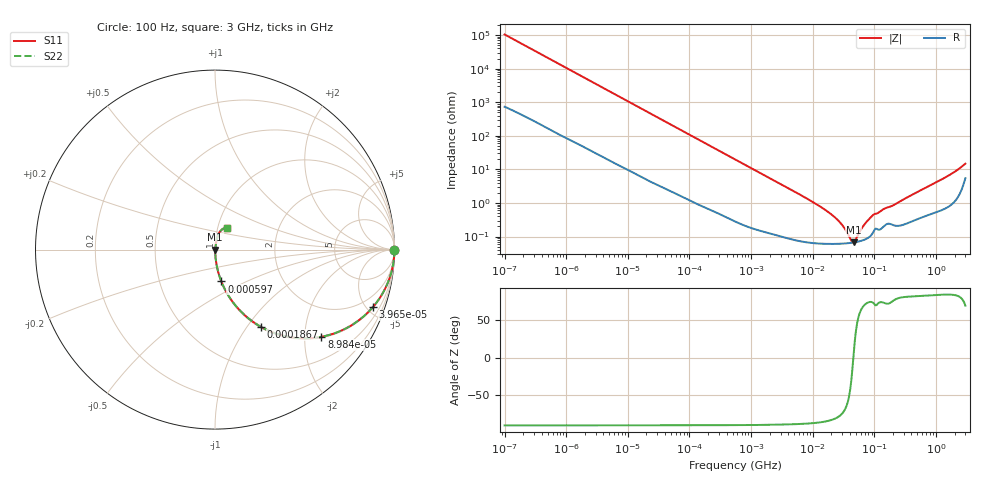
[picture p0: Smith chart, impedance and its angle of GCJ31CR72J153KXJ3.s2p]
!Murata Part Number: GCJ31CR72J153KXJ3
!These Parameters are Measured in Series Mode Connection
!Data Generated on Mar 13, 2026
!  o--ll--o
!Port1  Port2
!  o------o
!Operation Temp=25[degC], DC Bias Voltage=0[V]
!Freq. Start=100[Hz] Stop=3[GHz] 401[Steps]
# Hz S RI R 50
!Freq.(Hz) S11(Real) S11(Imag) S21(Real) S21(Imag) S12(Real) S12(Imag) S22(Real) S22(Imag)
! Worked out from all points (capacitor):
!   401 points, 100 Hz to 3 GHz, reference 50 ohm
!   read as one part in series: C = 15.2 nF near 109 Hz
!   lowest |Z| = 67 mohm at 46.12 MHz (marker M1)
!   series resonance near 45.61 MHz, so ESL is about 800 pH
!   S11 on the Smith chart (normalised r, x): 100 Hz: open; 39.66 kHz: 1.05, -5.45; 89.84 kHz: 1.03, -2.42; 186.7 kHz: 1.01, -1.17; 597 kHz: 1.01, -0.37; 3 GHz: 1.11, +0.28
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100  1 -0.000956  7.6e-06 0.000956  7.6e-06 0.000956  1 -0.000956
1788  0.9996 -0.0168  0.000425 0.0168  0.000425 0.0168  0.9996 -0.0168
9582  0.9913 -0.0885  0.00871 0.0885  0.00871 0.0885  0.9913 -0.0885
31977  0.9171 -0.271  0.0829 0.271  0.0829 0.271  0.9171 -0.271
39655  0.8788 -0.3214  0.1212 0.3214  0.1212 0.3214  0.8788 -0.3214
89839  0.5929 -0.4859  0.4071 0.4859  0.4071 0.4859  0.5929 -0.4859
186741  0.2572 -0.4311  0.7428 0.4311  0.7428 0.4311  0.2572 -0.4311
299821  0.121 -0.3197  0.879 0.3197  0.879 0.3197  0.121 -0.3197
547723  0.0413 -0.1921  0.9587 0.1921  0.9587 0.1921  0.0413 -0.1921
596961  0.0353 -0.1775  0.9647 0.1775  0.9647 0.1775  0.0353 -0.1775
1827928  0.00495 -0.0603  0.9951 0.0603  0.9951 0.0603  0.00495 -0.0603
9794414  0.000762 -0.0109  0.9992 0.0109  0.9992 0.0109  0.000762 -0.0109
2.418395e7  0.000617 -0.00335  0.9994 0.00335  0.9994 0.00335  0.000617 -0.00335
3.131008e7  0.000622 -0.0019  0.9994 0.0019  0.9994 0.0019  0.000622 -0.0019
4.231884e7  0.000652 -0.000371  0.9993 0.000371  0.9993 0.000371  0.000652 -0.000371
4.612319e7  0.000667 5.68e-05  0.9993 -5.68e-05  0.9993 -5.68e-05  0.000667 5.68e-05
5.026954e7  0.000686 0.000486  0.9993 -0.000486  0.9993 -0.000486  0.000686 0.000486
6.794454e7  0.000802 0.00206  0.9992 -0.00206  0.9992 -0.00206  0.000802 0.00206
8.79653e7  0.00109 0.00363  0.9989 -0.00363  0.9989 -0.00363  0.00109 0.00363
1.751444e8  0.00246 0.00723  0.9975 -0.00723  0.9975 -0.00723  0.00246 0.00723
1.324213e9  0.00922 0.0527  0.9908 -0.0527  0.9908 -0.0527  0.00922 0.0527
3e9  0.0677 0.1223  0.9323 -0.1223  0.9323 -0.1223  0.0677 0.1223
